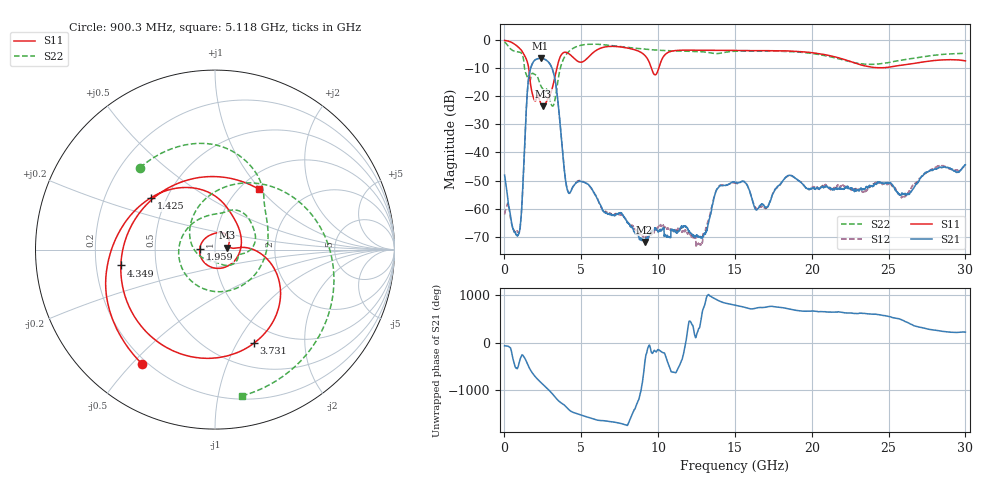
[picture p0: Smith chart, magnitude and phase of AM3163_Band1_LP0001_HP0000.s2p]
!Agilent Technologies,E8364B,MY43040894,A.07.50.67
!Agilent E8364B: A.07.50.67
!Date: Thursday, August 20, 2020 11:22:59
!Correction: S11(Full 2 Port(1,2))
!S21(Full 2 Port(1,2))
!S12(Full 2 Port(1,2))
!S22(Full 2 Port(1,2))
!S2P File: Measurements: S11, S21, S12, S22:
# Hz S  dB  R 50
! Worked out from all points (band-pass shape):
!   3201 points, 10 MHz to 30 GHz, reference 50 ohm
!   highest |S21| = -6.41 dB at 2.353 GHz (marker M1); lowest = -71.9 dB at 9.119 GHz (marker M2)
!   |S21| within 3 dB of the highest: 1.739 GHz to 3.055 GHz (1.316 GHz wide, 54.9 % of centre)
!   lowest |S11| = -23.5 dB at 2.522 GHz (marker M3), VSWR 1.14, Z = 57 + j1.29 ohm
!   |S11| at or under -10 dB: 1.581 GHz to 3.406 GHz (1.825 GHz wide, 73.2 % of centre); 9.568 GHz to 10.04 GHz (471.3 MHz wide, 4.81 % of centre)
!   |S22| runs from -23.5 to -0.6 dB; largest |S21 - S12| = 0.0034
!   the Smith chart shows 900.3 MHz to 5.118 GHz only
!   S11 on the Smith chart (normalised r, x): 900.3 MHz: 0.18, -0.53; 1.425 GHz: 0.41, +0.30; 1.959 GHz: 0.84, +0.01; 3.731 GHz: 0.77, -1.18; 4.349 GHz: 0.31, -0.08; 5.118 GHz: 1.21, +0.98
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1e7  -0.07 -8.8  -48.07 -65.4  -62.09 -26.4  -0.63 -28.4
4.5985e8  -0.76 -61.1  -65.00 173.5  -65.21 -121.9  -3.38 -147.8
9.003281e8  -2.44 -122.6  -69.17 -135.3  -68.54 -159.1  -4.17 132.4
1.425153e9  -6.76 141.0  -24.27 -31.5  -24.16 -31.7  -12.28 -68.2
1.95935e9  -21.40 176.9  -7.18 21.9  -7.18 21.9  -12.12 33.2
2.352969e9  -22.32 16.4  -6.41 -112.8  -6.41 -112.8  -16.06 -8.2
2.521662e9  -23.49 9.7  -6.57 -164.6  -6.57 -164.7  -17.35 -12.0
3.224553e9  -14.46 2.5  -12.30 -36.3  -12.32 -36.2  -22.66 -131.1
3.730634e9  -4.96 -67.3  -36.43 163.0  -36.43 163.9  -8.21 70.9
4.349178e9  -5.48 -170.4  -53.49 -9.4  -53.50 -10.5  -3.29 -14.4
5.014581e9  -7.81 72.8  -50.40 -86.4  -50.14 -86.2  -1.74 -72.1
5.117672e9  -7.62 53.9  -50.52 -97.0  -50.33 -96.4  -1.63 -79.6
6.373503e9  -2.61 -100.9  -60.39 159.4  -60.51 149.7  -1.56 -154.0
7.535616e9  -2.37 -177.8  -61.41 103.1  -62.11 95.9  -2.24 153.7
9.119462e9  -5.29 96.8  -71.93 -96.6  -70.03 -2.3  -3.18 91.7
1.000979e10  -10.50 116.0  -68.34 -144.1  -66.53 -21.9  -3.55 58.9
1.274638e10  -3.52 -5.0  -70.05 26.6  -72.67 174.8  -4.06 -33.8
1.5005e10  -3.64 -72.2  -50.61 67.9  -50.85 69.2  -3.92 -90.3
2.000958e10  -4.43 163.2  -52.76 -51.2  -52.44 -63.4  -4.70 136.7
2.275554e10  -8.03 60.1  -53.66 -104.3  -52.99 -105.0  -7.98 21.2
2.500479e10  -9.63 -62.2  -50.94 -166.1  -51.14 -163.3  -7.96 -92.0
3e10  -7.35 105.5  -44.36 -137.3  -44.37 -129.8  -4.65 102.4
